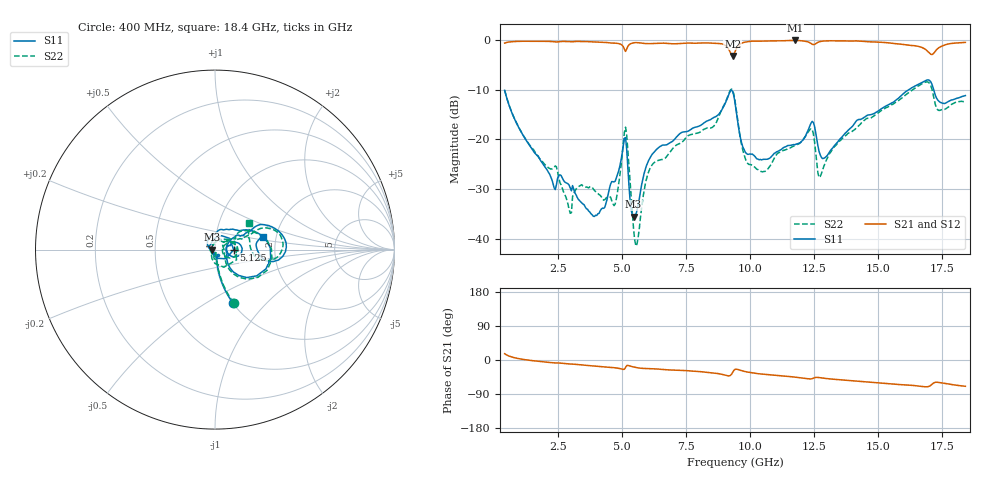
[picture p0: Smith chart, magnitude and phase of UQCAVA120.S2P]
!  Part Number  UQCAVA120
!  Description: RF capacitor  Mounting Orientation: Horizontal
!  Application:
# GHZ S DB R 50
! Freq  |S11|  S11 Ph  |S21|  S21 Ph  |S12|  S12 Ph  |S22|  S22 Ph
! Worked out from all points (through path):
!   401 points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, 400 MHz to 18.4 GHz, reference 50 ohm
!   highest |S21| = -0.04 dB at 11.74 GHz (marker M1); lowest = -3.2 dB at 9.31 GHz (marker M2)
!   group delay of S21, straight-line fit = 11.3 ps
!   lowest |S11| = -35.6 dB at 5.44 GHz (marker M3), VSWR 1.03, Z = 48.4 + j0.0459 ohm
!   |S11| at or under -10 dB: start of sweep to 16.18 GHz; 17.16 GHz to end of sweep
!   |S22| runs from -41.5 to -8.4 dB; largest |S21 - S12| = 0.0035
!   S11 on the Smith chart (normalised r, x): 400 MHz: 1.00, -0.66; 5.125 GHz: 1.23, -0.00; 18.4 GHz: 1.71, +0.26
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0.4  -10.10 -71.5  -0.57 16.5  -0.55 16.5  -10.07 -70.7
2.29  -28.89 -74.7  -0.28 -7.4  -0.26 -7.4  -25.86 -78.0
2.92  -29.23 -75.5  -0.29 -10.5  -0.27 -10.6  -34.14 -88.1
3.415  -32.82 -93.1  -0.25 -13.1  -0.23 -13.2  -29.14 -92.3
4  -35.34 -125.0  -0.34 -16.6  -0.32 -16.6  -30.77 -125.5
4.675  -28.58 130.0  -0.57 -20.2  -0.55 -20.3  -33.36 136.4
5.125  -19.63 -0.5  -2.25 -19.5  -2.24 -19.6  -17.54 -25.7
5.44  -35.62 178.4  -0.52 -18.4  -0.50 -18.5  -38.24 -146.1
5.575  -34.29 167.3  -0.48 -20.3  -0.46 -20.4  -41.05 -172.2
5.98  -24.79 137.8  -0.68 -22.5  -0.67 -22.7  -27.25 83.8
6.43  -21.59 103.4  -0.59 -24.1  -0.59 -24.2  -24.18 42.9
8.95  -13.43 30.9  -0.83 -38.9  -0.85 -39.1  -13.28 28.5
9.31  -10.35 -20.7  -3.19 -32.4  -3.21 -32.6  -10.10 -21.5
9.4  -12.56 -41.4  -2.32 -24.8  -2.33 -25.0  -12.21 -42.3
9.94  -23.00 -19.2  -0.27 -32.4  -0.28 -32.5  -25.05 -16.6
11.74  -21.08 15.5  -0.04 -45.1  -0.04 -45.2  -21.32 30.4
12.415  -16.37 2.1  -0.79 -49.3  -0.80 -49.4  -18.00 -10.0
12.73  -23.15 -11.3  -0.25 -46.8  -0.26 -46.9  -27.48 4.7
15.43  -12.92 28.1  -0.54 -62.9  -0.55 -62.8  -13.26 23.1
16.87  -8.09 7.9  -1.96 -70.8  -1.98 -70.7  -8.40 7.3
17.365  -12.31 -3.8  -1.50 -59.2  -1.50 -59.2  -14.16 6.6
18.4  -11.16 14.5  -0.43 -69.3  -0.45 -69.3  -12.37 37.4
